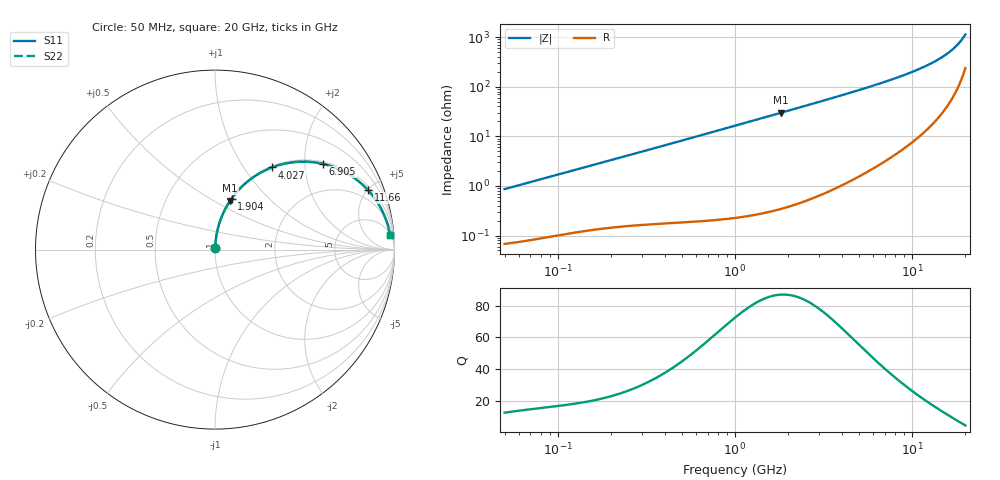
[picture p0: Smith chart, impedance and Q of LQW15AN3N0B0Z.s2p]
!Murata Part Number: LQW15AN3N0B0Z
!These Parameters are Measured in Series Mode Connection
!  o--[Z]--o
!Port1  Port2
!  o-------o
!Freq. Start=50[MHz] Stop=20[GHz], 401[Steps]
# Hz S RI R 50
!Freq.(Hz) S11(Real) S11(Imag) S21(Real) S21(Imag) S12(Real) S12(Imag) S22(Real) S22(Imag)
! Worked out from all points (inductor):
!   401 points, 50 MHz to 20 GHz, reference 50 ohm
!   read as one part in series: L = 2.73 nH near 51.52 MHz
!   highest Q = 86.9 at 1.821 GHz (marker M1), where L = 2.62 nH
!   S11 on the Smith chart (normalised r, x): 50 MHz: 1.00, +0.02; 1.904 GHz: 1.01, +0.63; 4.027 GHz: 1.02, +1.35; 6.905 GHz: 1.06, +2.46; 11.66 GHz: 1.24, +5.03; 20 GHz: 6, +22
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5e7  0.000751 0.00859  0.9992 -0.00859  0.9992 -0.00859  0.000751 0.00859
1.364002e8  0.00173 0.0228  0.9983 -0.0228  0.9983 -0.0228  0.00173 0.0228
3.721004e8  0.00543 0.0607  0.9946 -0.0607  0.9946 -0.0607  0.00543 0.0607
6.285508e8  0.0124 0.1015  0.9876 -0.1015  0.9876 -0.1015  0.0124 0.1015
1e9  0.0282 0.1588  0.9718 -0.1588  0.9718 -0.1588  0.0282 0.1588
1.390315e9  0.0517 0.2155  0.9483 -0.2155  0.9483 -0.2155  0.0517 0.2155
1.820564e9  0.0848 0.2728  0.9152 -0.2728  0.9152 -0.2728  0.0848 0.2728
1.904239e9  0.0919 0.2832  0.9081 -0.2832  0.9081 -0.2832  0.0919 0.2832
2.728004e9  0.1724 0.3716  0.8276 -0.3716  0.8276 -0.3716  0.1724 0.3716
3.314454e9  0.2366 0.4183  0.7634 -0.4183  0.7634 -0.4183  0.2366 0.4183
4.026975e9  0.3171 0.4578  0.6829 -0.4578  0.6829 -0.4578  0.3171 0.4578
5.352748e9  0.4599 0.4889  0.5401 -0.4889  0.5401 -0.4889  0.4599 0.4889
6.905011e9  0.6007 0.4777  0.3993 -0.4777  0.3993 -0.4777  0.6007 0.4777
7.442007e9  0.6418 0.4664  0.3582 -0.4664  0.3582 -0.4664  0.6418 0.4664
9.457416e9  0.7639 0.4074  0.2361 -0.4074  0.2361 -0.4074  0.7639 0.4074
1.166392e10  0.8522 0.3319  0.1478 -0.3319  0.1478 -0.3319  0.8522 0.3319
1.375312e10  0.9061 0.2615  0.0939 -0.2615  0.0939 -0.2615  0.9061 0.2615
1.597544e10  0.9425 0.1921  0.0575 -0.1921  0.0575 -0.1921  0.9425 0.1921
1.774144e10  0.9609 0.1416  0.0391 -0.1416  0.0391 -0.1416  0.9609 0.1416
1.855685e10  0.967 0.1196  0.033 -0.1196  0.033 -0.1196  0.967 0.1196
1.940974e10  0.972 0.0974  0.028 -0.0974  0.028 -0.0974  0.972 0.0974
2e10  0.9748 0.0826  0.0252 -0.0826  0.0252 -0.0826  0.9748 0.0826
